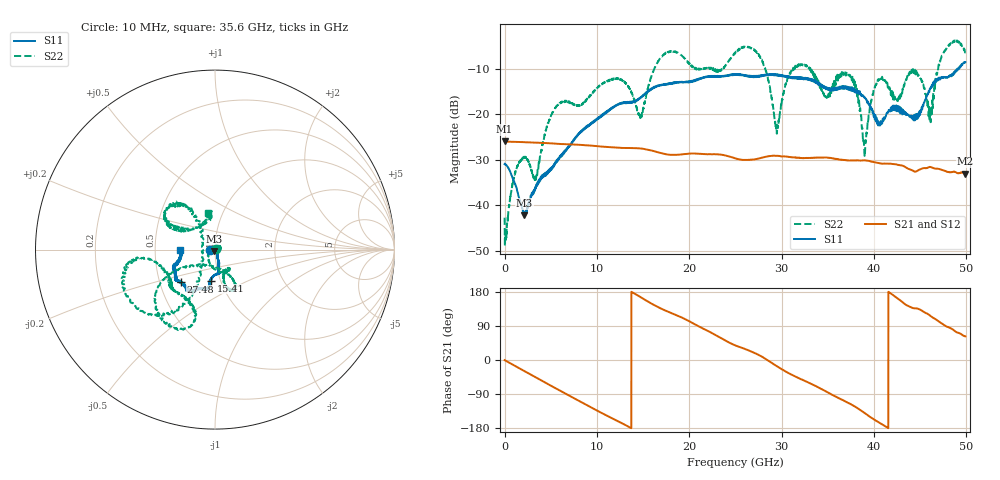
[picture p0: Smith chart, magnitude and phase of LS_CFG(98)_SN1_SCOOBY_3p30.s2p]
!Keysight Technologies,N5245B,MY58422026,A.13.80.08
!Date: Thursday, March 19, 2020 23:57:52
!Correction: S11(Full 2 Port(1,2))
!S21(Full 2 Port(1,2))
!S12(Full 2 Port(1,2))
!S22(Full 2 Port(1,2))
!S2P File: Measurements: S11, S21, S12, S22:
# Hz S DB R 50.0
!freq dBS11 angS11 dBS21 angS21 dBS12 angS12 dBS22 angS22
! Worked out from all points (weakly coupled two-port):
!   4991 points, 10 MHz to 49.91 GHz, reference 50 ohm
!   highest |S21| = -25.96 dB at 10 MHz (marker M1); lowest = -33.0 dB at 49.91 GHz (marker M2)
!   lowest |S11| = -42.2 dB at 2.14 GHz (marker M3), VSWR 1.02, Z = 49.7 - j0.691 ohm
!   |S11| at or under -10 dB: start of sweep to 49.02 GHz; 49.04555 GHz to 49.11026 GHz (64.72 MHz wide, 0.132 % of centre); 49.18497 GHz to 49.21101 GHz (26.04 MHz wide, 0.0529 % of centre)
!   |S22| runs from -49.0 to -3.7 dB; largest |S21 - S12| = 0.00048
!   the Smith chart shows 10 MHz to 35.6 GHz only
!   S11 on the Smith chart (normalised r, x): 10 MHz: 0.95, -0.01; 15.41 GHz: 0.90, -0.32; 27.48 GHz: 0.64, -0.25; 35.6 GHz: 0.68, -0.01
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1e7  -30.95 -174.5  -25.96 -0.3  -25.96 -0.3  -42.76 7.9
2.14e9  -42.19 -116.4  -26.12 -29.1  -26.11 -29.1  -29.41 22.8
3.33e9  -36.01 -67.0  -26.22 -45.0  -26.21 -45.0  -33.91 130.8
5.38e9  -30.88 -63.1  -26.42 -72.7  -26.41 -72.6  -18.97 -88.0
8.33e9  -23.88 -73.2  -26.73 -111.6  -26.72 -111.5  -17.82 -62.8
1.541e10  -15.18 -97.7  -27.71 156.0  -27.71 156.1  -15.31 -146.5
1.665e10  -13.74 -99.1  -28.37 139.2  -28.36 139.3  -8.26 -145.4
1.985e10  -12.83 -106.6  -28.68 104.3  -28.67 104.4  -8.59 -106.4
2.496e10  -11.28 -125.4  -29.64 38.9  -29.63 39.1  -6.55 -171.0
2.748e10  -11.71 -136.8  -29.76 13.9  -29.76 14.1  -6.72 -127.9
2.947e10  -11.19 -142.7  -29.12 -16.0  -29.12 -15.7  -23.39 -176.2
3.103e10  -11.78 -149.9  -29.43 -38.1  -29.44 -37.8  -10.40 125.7
3.328e10  -12.40 -160.4  -29.56 -63.9  -29.56 -63.5  -10.62 153.0
3.56e10  -14.26 -178.4  -29.73 -93.5  -29.67 -93.1  -13.92 101.3
3.77e10  -14.86 171.0  -30.13 -119.5  -30.07 -119.6  -12.19 131.6
3.902e10  -16.29 168.1  -30.12 -140.1  -30.10 -140.4  -28.39 -113.1
4.021e10  -21.45 153.6  -30.59 -159.8  -30.57 -160.0  -13.44 -9.0
4.16e10  -19.11 100.1  -30.85 179.5  -30.88 179.5  -14.16 22.3
4.437e10  -20.24 57.6  -32.58 136.3  -32.61 136.4  -10.39 -15.0
4.614e10  -14.19 5.7  -31.58 116.0  -31.60 116.2  -21.42 -51.4
4.757e10  -11.77 5.3  -32.37 92.8  -32.39 92.8  -6.27 -80.4
4.991e10  -8.49 -14.0  -33.04 62.3  -33.06 62.4  -6.29 -28.7
